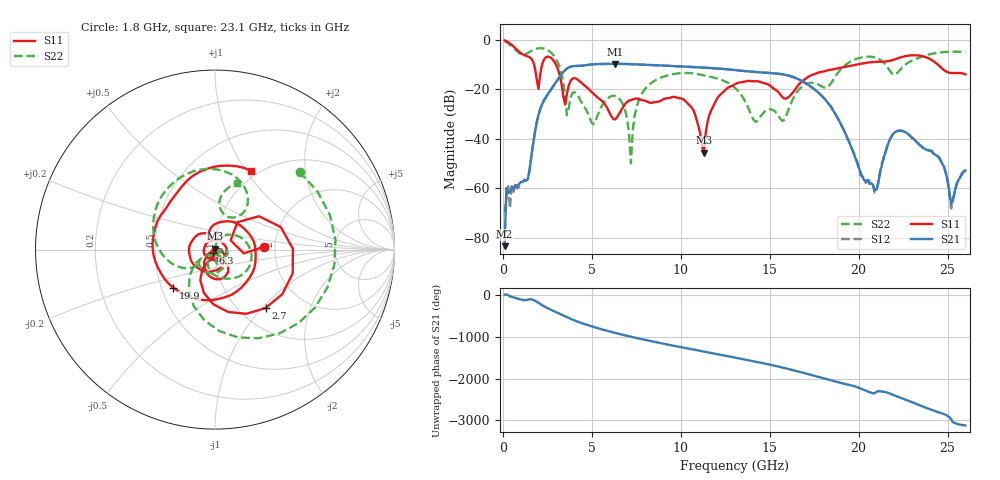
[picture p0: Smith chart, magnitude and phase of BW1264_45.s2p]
!Keysight Technologies,N5245B,MY57181159,A.13.60.06
!Date: Friday, December 18, 2020 23:54:27
!Correction: S11(Full 2 Port(1,2))
!S21(Full 2 Port(1,2))
!S12(Full 2 Port(1,2))
!S22(Full 2 Port(1,2))
!S2P File: Measurements: S11, S21, S12, S22:
# Hz S  dB  R 50
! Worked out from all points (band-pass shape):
!   260 points, 100 MHz to 26 GHz, reference 50 ohm
!   highest |S21| = -9.79 dB at 6.3 GHz (marker M1); lowest = -83.3 dB at 100 MHz (marker M2)
!   |S21| within 3 dB of the highest: 3.439 GHz to 13.73 GHz (10.29 GHz wide, 120 % of centre)
!   lowest |S11| = -45.6 dB at 11.3 GHz (marker M3), VSWR 1.01, Z = 50.2 + j0.476 ohm
!   |S11| at or under -10 dB: 1.747 GHz to 2.212 GHz (464.4 MHz wide, 23.5 % of centre); 2.977 GHz to 19.93 GHz (16.95 GHz wide, 148 % of centre); 24.44 GHz to end of sweep
!   |S22| runs from -49.9 to -0.5 dB; largest |S21 - S12| = 0.00051
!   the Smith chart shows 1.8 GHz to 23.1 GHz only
!   S11 on the Smith chart (normalised r, x): 1.8 GHz: 1.75, +0.06; 2.7 GHz: 1.31, -1.05; 6.3 GHz: 0.97, -0.04; 19.9 GHz: 0.58, -0.27; 23.1 GHz: 0.93, +1.06
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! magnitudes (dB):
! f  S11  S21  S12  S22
! 100 MHz  -0.4  -83.3  -69.6  -0.5
! 200 MHz  -0.6  -59.9  -64.0  -1.0
! 1.4 GHz  -6.8  -56.3  -56.1  -5.4
! 1.8 GHz  -11.2  -37.5  -37.5  -3.9
! 2.7 GHz  -7.3  -20.2  -20.2  -5.2
! 3.6 GHz  -22.0  -11.7  -11.7  -30.5
! 4.5 GHz  -17.9  -10.5  -10.5  -26.3
! 6.3 GHz  -32.2  -9.8  -9.8  -22.7
! 7.2 GHz  -24.4  -9.9  -9.9  -49.9
! 7.6 GHz  -23.9  -10.0  -10.0  -25.3
! 8.8 GHz  -24.9  -10.4  -10.4  -15.6
! 10.6 GHz  -27.3  -11.0  -11.0  -13.6
! 11.3 GHz  -45.6  -11.3  -11.3  -14.4
! 13.1 GHz  -17.8  -12.3  -12.3  -19.8
! 15.7 GHz  -23.1  -14.0  -14.0  -32.8
! 17.4 GHz  -14.2  -19.4  -19.4  -17.4
! 19.9 GHz  -10.0  -49.3  -49.0  -7.7
! 20.9 GHz  -9.1  -60.7  -61.7  -7.2
! 21.7 GHz  -8.6  -41.1  -41.1  -12.0
! 23.1 GHz  -6.3  -40.0  -40.2  -8.2
! 25.2 GHz  -13.5  -66.3  -68.1  -4.9
! 26 GHz  -14.0  -52.7  -53.1  -4.9
